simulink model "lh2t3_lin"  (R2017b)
settings: Solver=ode45  StartTime=0.0  StopTime=10.0  RelTol=1e-3  EnableMultiTasking=on
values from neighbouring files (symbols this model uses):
  amp = 1.8    [lh2t3.m]
  i0 = -R/(2*k)+sqrt(R^2/(4*k^2)+u0/k)    [lh2t3.m]
  k = 1    [lh2t3.m]
  L = 1    [lh2t3.m]
  R = 1    [lh2t3.m]
  u0 = 4    [lh2t3.m]

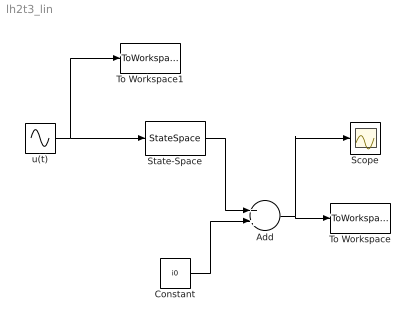
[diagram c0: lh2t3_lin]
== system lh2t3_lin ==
  Add : Sum
  Constant : Constant  Value=i0
  Scope : Scope
  State-Space : StateSpace  A=-R/L-2*k/L*(-R/(2*k)+sqrt(R^2/(4*k^2)+u0/k))  B=1/L  D=0  InitialCondition=0
  To Workspace : ToWorkspace  VariableName=i_lin  SampleTime=-1
  To Workspace1 : ToWorkspace  VariableName=u_lin  SampleTime=-1
  u(t) : Sin  Amplitude=amp  SampleTime=0
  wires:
  u(t)/1 -> State-Space/1, To Workspace1/1
  State-Space/1 -> Add/1
  Constant/1 -> Add/2
  Add/1 -> To Workspace/1, Scope/1
